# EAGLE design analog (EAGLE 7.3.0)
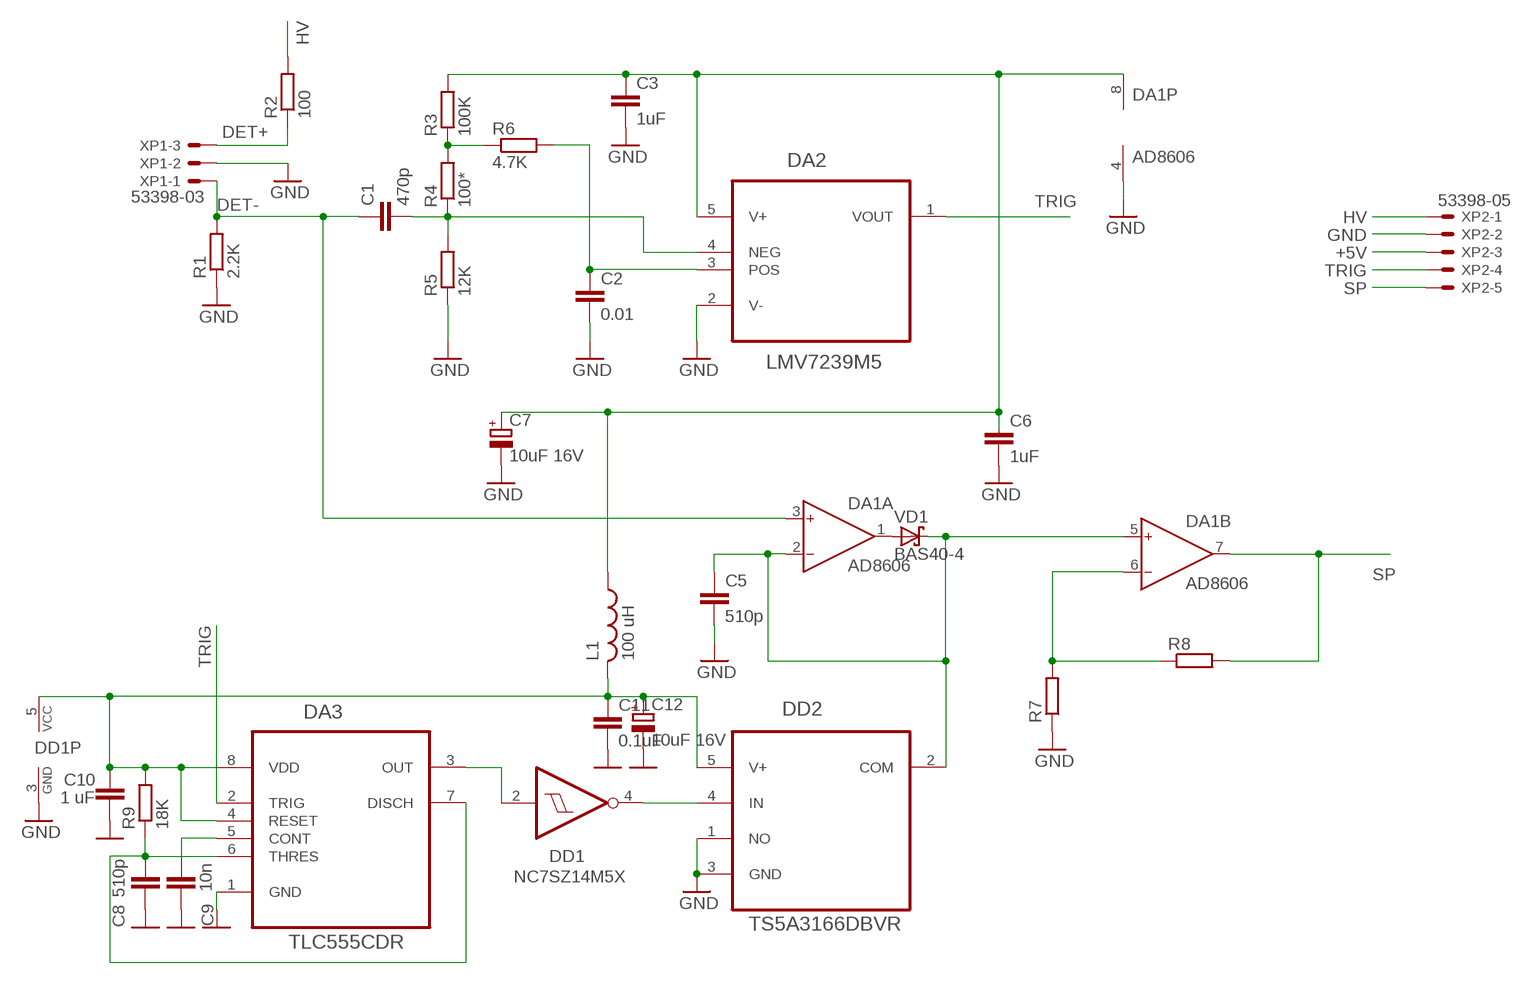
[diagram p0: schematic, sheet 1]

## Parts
C1  470p  C-EUC0603  [C0603]
C2  0.01  C-EUC0603  [C0603]
C3  1uF  C-EUC0805  [C0805]
C5  510p  C-EUC1206  [C1206]
C6  1uF  C-EUC0805  [C0805]
C7  10uF 16V  CPOL-EUSMCA  [SMC_A]
C8  510p  C-EUC0603K  [C0603K]
C9  10n  C-EUC0603K  [C0603K]
C10  1 uF  C-EUC0805  [C0805]
C11  0.1uF  C-EUC0805  [C0805]
C12  10uF 16V  CPOL-EUSMCA  [SMC_A]
DA1  AD8606  AD8607R  [SO8]
DA2  LMV7239M5  [SOT95P284X119-5N]
DA3  TLC555CDR  [SOIC127P600X175-8N]
DD1  NC7SZ14M5X  [SOT23-5]
DD2  TS5A3166DBVR  [SOT95P280X145-5N]
L1  100 uH  L-USL1812  [L1812]
R1  2.2K  R-EU_R0603  [R0603]
R2  100  R-EU_R0603  [R0603]
R3  100K  R-EU_R0603  [R0603]
R4  100*  R-EU_R0603  [R0603]
R5  12K  R-EU_R0603  [R0603]
R6  4.7K  R-EU_R0603  [R0603]
R7  R-EU_R0603  [R0603]
R8  R-EU_R0603  [R0603]
R9  18K  R-EU_R0603  [R0603]
VD1  BAS40-4  BAT54  [SOT23]
XP1  53398-03  [53398-03]
XP2  53398-05  [53398-05]

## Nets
+5V: C3.1 C6.1 C7.+ DA1.8(P:V+) DA2.5(V+) L1.1 R3.2 XP2.3
+5VD: C10.1 C11.1 C12.+ DA3.4(RESET) DA3.8(VDD) DD1.5(VCC) DD2.5(V+) L1.2 R9.2
DET+: R2.1 XP1.3
DET-: C1.1 DA1.3(A:IN+) R1.2 XP1.1
GND: C2.2 C3.2 C5.2 C6.2 C7.- C8.2 C9.2 C10.2 C11.2 C12.- DA1.4(P:V-) DA2.2(V-) DA3.1(GND) DD1.3(GND) DD2.1(NO) DD2.3(GND) R1.1 R5.1 R7.1 XP1.2 XP2.2
HV: R2.2 XP2.1
N$3: C1.2 DA2.4(NEG) R4.1 R5.2
N$4: R3.1 R4.2 R6.1
N$5: C2.1 DA2.3(POS) R6.2
N$7: DA1.1(A:OUT) VD1.1(A)
N$8: C5.1 DA1.2(A:IN-) DA1.5(B:IN+) DD2.2(COM) VD1.3(C)
N$9: DD1.4(O) DD2.4(IN)
N$10: DA3.3(OUT) DD1.2(I)
N$11: DA1.6(B:IN-) R7.2 R8.1
N$12: C9.1 DA3.5(CONT)
N$13: C8.1 DA3.6(THRES) DA3.7(DISCH) R9.1
SP: DA1.7(B:OUT) R8.2 XP2.5
TRIG: DA2.1(VOUT) DA3.2(TRIG) XP2.4

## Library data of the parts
C1-C3 C5 C6 C8-C11 = resistor:C-EU: CAPACITOR, European symbol
C7 C12 = resistor:CPOL-EU: POLARIZED CAPACITOR, European symbol
DA1 = analog-devices:AD8607: Precision Micropower, Low Noise CMOS, Rail-to-Rail Input/Output Operational Amplifiers Source: http://www.analog.com/static/imported-files/data_sheets/AD8603_8607_8609.pdf; MPN: AD8607ARMZ-R2; OC_FARNELL: 1651293; OC_NEWARK: 19M8927
DA2 = LMV7239M5:LMV7239M5: Comparator; AVAILABILITY: Good; DESCRIPTION: 75 nsec, Ultra Low Pwr, Low Voltage, Rail-to-Rail Input Comparator w/ Open-Drain/Push-Pull Output 5-SOT-23 -40 to 85; MF: Texas Instruments; MP: LMV7239M5; PACKAGE: SOT-23 Texas Instruments; PRICE: 1.72 USD
DA3 = Texas Instruments_By_element14_Batch_1:TLC555CDR: TIMER; MPN: TLC555CDR; OC_FARNELL: 8454426; OC_NEWARK: 35C2153; PACKAGE: SOIC-8; SUPPLIER: TI
DD1 = 74xx-little-us:NC7SZ14: TinyLogic(R) UHS Inverter with Schmitt Trigger Input Source: http://www.fairchildsemi.com/ds/NC/NC7SZ14.pdf
DD2 = Texas Instruments_By_element14_Batch_1:TS5A3166DBVR: .9- OHM SPST ANALOG SWITCH; MPN: TS5A3166DBVR; OC_FARNELL: 1755409; OC_NEWARK: 08K5004; PACKAGE: SOT-23-5; SUPPLIER: Texas Instruments
L1 = resistor:L-US: INDUCTOR, American symbol
R1-R9 = resistor:R-EU_: RESISTOR, European symbol
VD1 = diode:BAT54: Schottky Diodes
XP1 = con-molex:53?-03: CONNECTOR wire to board 1.25 mm (.049 inch) pitch header; OC_FARNELL: unknown; OC_NEWARK: unknown
XP2 = con-molex:53?-05: CONNECTOR wire to board 1.25 mm (.049 inch) pitch header; OC_FARNELL: 1125354; OC_NEWARK: unknown

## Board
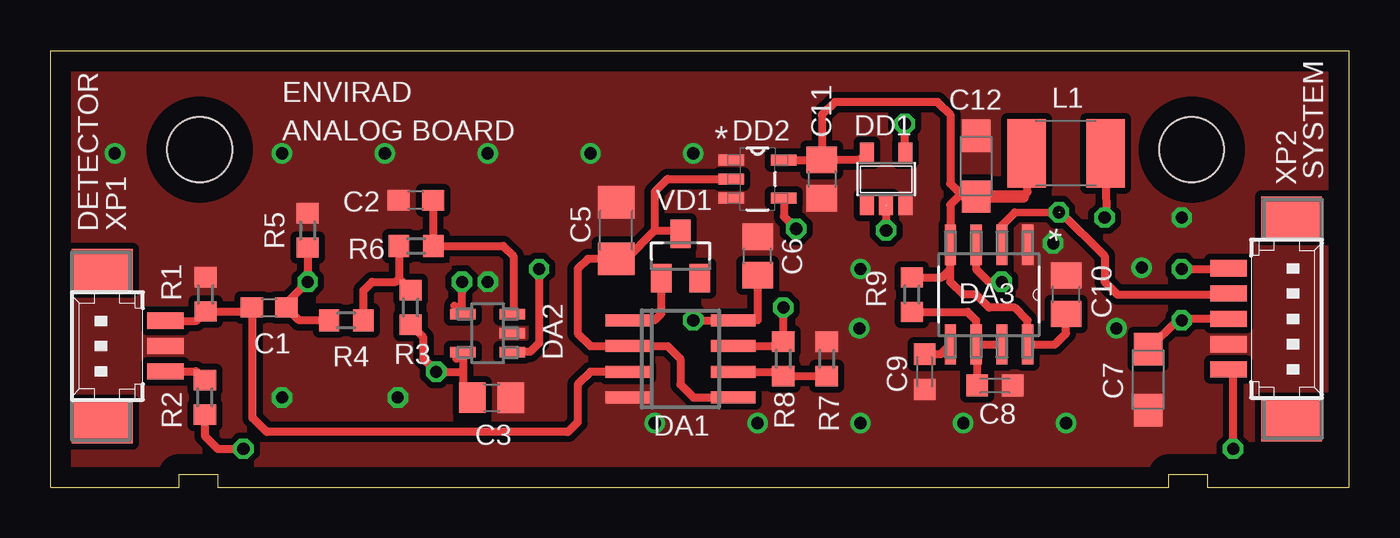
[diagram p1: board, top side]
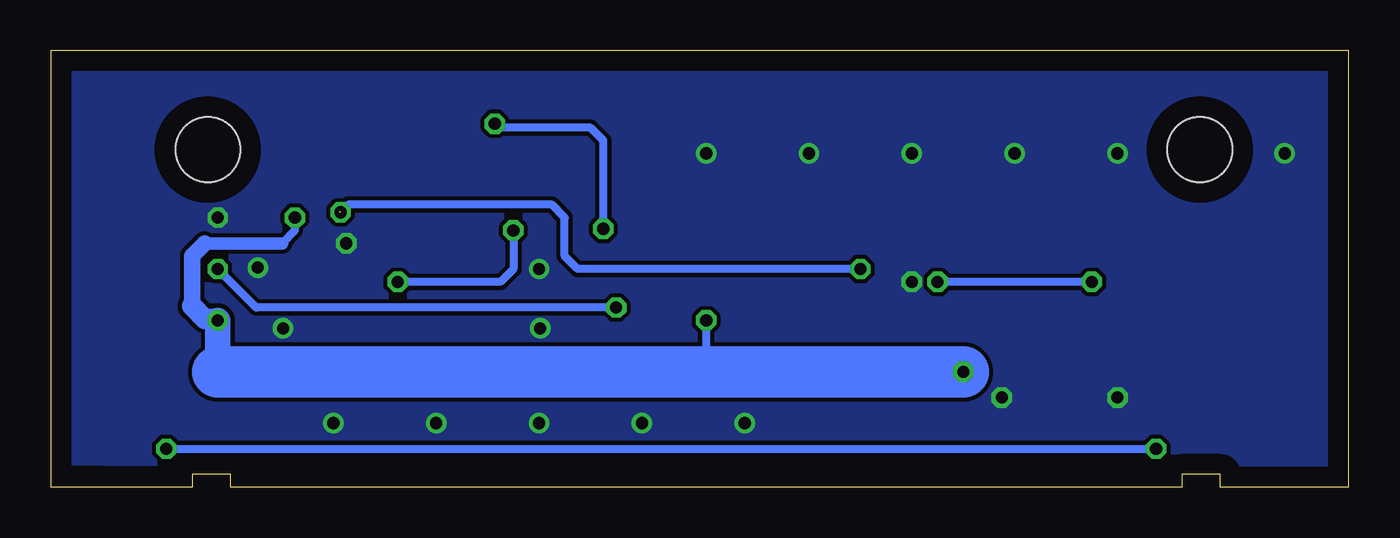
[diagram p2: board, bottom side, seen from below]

Size 64.13 x 21.59 mm. Coordinates in mm from the lower left corner, seen from the top.
Outline: 0,21.59 64.13,21.59 64.13,0 57.15,0 57.15,0.63 55.25,0.63 55.25,0 8.26,0 8.26,0.63 6.35,0.63 6.35,0 0,0 0,21.59
Copper layers (1*16): Top 0.035mm / dielectric 1.5mm / Bottom 0.035mm
Design rules "default *": minimum track width 8mil, minimum drill 12mil, track to track 8mil, track to pad 8mil, pad to pad 8mil, via to via 8mil, smd to smd 8mil, copper to edge 40mil, drill to drill 8mil, minimum pad ring 10mil, minimum via ring 8mil, stop-mask expansion 4mil, vias tented up to drill 32mil, thermal gap 10mil
Holes 3.2 mm at 7.37,16.7 56.37,16.7

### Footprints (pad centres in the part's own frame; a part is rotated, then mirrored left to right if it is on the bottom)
C0603 = smd 1.1 x 1: 1 -0.85,0; 2 0.85,0
C0805 = smd 1.3 x 1.5: 1 -0.95,0; 2 0.95,0
C1206 = smd 1.6 x 1.8: 1 -1.4,0; 2 1.4,0
SMC_A = smd 1.6 x 1.4: + -1.5,0; - 1.5,0
C0603K = smd 1.05 x 1.08: 1 -0.875,0; 2 0.875,0
SO8 = smd 0.6 x 2.2: 1 -1.905,-2.6; 2 -0.635,-2.6; 3 0.635,-2.6; 4 1.905,-2.6; 5 1.905,2.6; 6 0.635,2.6; 7 -0.635,2.6; 8 -1.905,2.6
SOT95P284X119-5N = smd 1.27 x 0.533: 1 -1.219,0.94; 2 -1.219,0; 3 -1.219,-0.94; 4 1.219,-0.94; 5 1.219,0.94
SOIC127P600X175-8N = smd 1.981 x 0.559: 1 -2.464,1.905; 2 -2.464,0.635; 3 -2.464,-0.635; 4 -2.464,-1.905; 5 2.464,-1.905; 6 2.464,-0.635; 7 2.464,0.635; 8 2.464,1.905
SOT23-5 = smd 0.69 x 0.99: 1 -0.95,-1.29; 2 0,-1.29; 3 0.95,-1.29; 4 0.95,1.3; 5 -0.95,1.3
SOT95P280X145-5N = smd 1.27 x 0.559: 1 -1.295,0.94; 2 -1.295,0; 3 -1.295,-0.94; 4 1.295,-0.94; 5 1.295,0.94
L1812 = smd 1.9 x 3.4: 1 -1.95,0; 2 1.95,0
R0603 = smd 1 x 1.1: 1 -0.85,0; 2 0.85,0
SOT23 = smd 1 x 1.4: 1 -0.95,-1.1; 2 0.95,-1.1; 3 0,1.1
53398-03 = smd 0.8 x 1.8: 1 1.25,-2.5; 2 0,-2.5; 3 -1.25,-2.5 | smd 2.1 x 3: S1 3.75,0.625; S2 -3.75,0.625
53398-05 = smd 0.8 x 1.8: 1 2.5,-2.5; 2 1.25,-2.5; 3 0,-2.5; 4 -1.25,-2.5; 5 -2.5,-2.5 | smd 2.1 x 3: S1 5,0.625; S2 -5,0.625

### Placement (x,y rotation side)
C1  10.79,8.89 0 top
C2  18.04,14.19 180 top
C3  21.79,4.44 0 top
C5  27.94,12.7 90 top
C6  34.93,11.43 90 top
C7  54.21,5.33 270 top
C8  46.65,5.03 0 top
C9  43.18,5.71 270 top
C10  50.16,9.52 90 top
C11  38.1,15.24 270 top
C12  45.72,15.88 90 top
DA1  31.11,6.35 270 top
DA2  21.59,7.62 180 top
DA3  46.36,9.52 270 top
DD1  41.27,15.24 0 top
DD2  34.93,15.24 0 top
L1  50.16,16.51 180 top
R1  7.65,9.54 270 top
R2  7.62,4.45 270 top
R3  17.78,8.89 270 top
R4  14.61,8.25 0 top
R5  12.7,12.7 270 top
R6  18.06,11.93 0 top
R7  38.34,6.35 270 top
R8  36.2,6.35 90 top
R9  42.55,9.52 90 top
VD1  31.11,11.43 0 top
XP1  3.17,6.98 90 top
XP2  60.68,8.33 270 top

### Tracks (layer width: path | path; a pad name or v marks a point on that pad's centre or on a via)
+5V  (via drill 0.6)
  Top 0.406: 20.04,6.35 DA2.5 20.37,5.71 | 20.37,5.71 20.37,4.91 C3.1 | C6.1 34.93,8.25 DA1.8 v31.75,8.25 | XP2.3 55.81,8.33 | C7.+ 55.72,8.33 55.81,8.33 | L1.1 52.16,13.43 v52.07,13.34 | 20.37,5.71 v19.05,5.71 18.41,6.35 18.41,7.41 R3.2 | 55.81,8.33 v55.88,8.25
  Bottom 0.406: v52.07,13.34 52.07,12.7 52.71,12.06 | 55.95,8.33 v55.88,8.25 | v31.75,8.25 31.75,5.71
  Bottom 0.61: 52.71,12.06 56.52,12.06
  Bottom 0.813: 56.52,12.06 57.15,11.43 57.15,8.96
  Bottom 1.016: 57.15,8.96 56.52,8.33 55.95,8.33
  Bottom 1.27: v55.88,8.25 55.88,5.71
  Bottom 2.54: 55.88,5.71 31.75,5.71 v19.05,5.71
+5VD
  Top 0.406: C12.+ 45.09,14.38 | 45.09,14.38 44.86,14.38 44.45,13.97 DA3.4 44.45,10.79 | R9.2 44.03,10.38 44.45,10.79 | C10.1 50.16,7.62 49.61,7.06 DA3.8 48.26,8.25 47.62,8.89 46.36,8.89 45.72,9.52 45.09,9.52 44.45,10.16 44.45,10.79 | 45.09,14.38 44.45,15.01 44.45,18.41 43.82,19.05 38.73,19.05 38.1,18.41 C11.1 | DD2.5 C11.1 | C11.1 39.98,16.19 DD1.5 | 48.03,14.38 48.26,14.6 48.26,15.78 L1.2
  Top 0.61: C12.+ 48.03,14.38
DET+
  Top 0.406: XP1.3 7.18,5.73 R2.1
DET-
  Top 0.406: XP1.1 7.2,8.23 R1.2 9.75,8.69 C1.1 9.98,8.86 9.98,3.43 10.68,2.73 25.55,2.73 26.04,3.22 26.04,5.08 26.67,5.71 DA1.3
GND  (via drill 0.6)
  other vias: 3.17,16.51 11.43,4.45 49.53,12.06 21.59,10.16 11.43,16.51 16.51,16.51 21.59,16.51 26.67,16.51 31.75,16.51 29.84,3.17 34.93,3.17 40.01,3.17 45.09,3.17 50.16,3.17 40.01,10.79 39.95,7.86 52.65,7.86 53.9,10.86 55.88,13.34 17.14,4.45
  pour Bottom: 0,20.95 0,0.63 64.13,1.27 64.13,20.95
  pour Top (isolate 0.305, no thermals): 0,20.95 64.13,20.95 64.13,1.27 0,0.63
HV  (via drill 0.6)
  Top 0.406: v58.42,1.91 58.42,5.59 XP2.1 | R2.2 7.62,2.54 8.26,1.91 v9.53,1.91
  Bottom 0.406: v58.42,1.91 v9.53,1.91
N$3  (via drill 0.6)
  Top 0.406: 19.95,8.98 20.18,8.75 | 20.18,8.75 DA2.4 | v20.32,10.16 20.32,8.89 20.18,8.75 | R5.2 v12.7,10.16 11.43,8.89 C1.2 12.28,8.25 R4.1
  Bottom 0.406: v12.7,10.16 v20.32,10.16
N$4
  Top 0.406: R6.1 17.21,10.31 | 17.21,10.31 R3.1 | R4.2 15.46,9.74 15.88,10.16 17.05,10.16 17.21,10.31
N$5
  Top 0.406: C2.1 18.89,11.95 R6.2 22.36,11.93 22.86,11.43 22.86,8.61 DA2.3
N$7
  Top 0.406: VD1.1 30.16,8.57 29.84,8.25 DA1.1
N$8
  Top 0.406: DA1.5 31.75,4.45 31.11,5.08 31.11,6.35 30.48,6.98 DA1.2 26.67,6.98 26.04,7.62 26.04,10.79 26.54,11.3 C5.1 28.44,11.3 29.84,12.7 | 29.84,12.7 30.94,12.7 VD1.3 | 29.84,12.7 29.84,14.6 30.48,15.24 DD2.2
N$9  (via drill 0.6)
  Top 0.406: v42.19,17.97 42.19,16.57 DD1.4 | DD2.4 36.22,13.39 v36.83,12.78
  Bottom 0.406: v36.83,12.78 36.83,17.15 37.47,17.78 42,17.78 v42.19,17.97
N$10  (via drill 0.6)
  Top 0.406: DA3.3 45.72,10.79 46.36,10.16 v46.99,10.16 | DD1.2 v41.27,12.7
  Bottom 0.406: v41.27,12.7 41.27,10.79 41.91,10.16 v46.99,10.16
N$11
  Top 0.406: DA1.6 35.98,5.71 R8.1 R7.2
N$12
  Top 0.406: C9.1 43.98,6.59 DA3.5
N$13
  Top 0.406: DA3.6 DA3.7 | C8.1 45.77,7.01 DA3.6 | R9.1 45.3,8.67 45.72,8.25 DA3.6
SP  (via drill 0.6)
  Top 0.406: DA1.7 35.98,6.98 R8.2 v36.2,8.89 | v55.88,10.79 58.15,10.79 XP2.5
  Bottom 0.406: v36.2,8.89 53.98,8.89 v55.88,10.79
TRIG  (via drill 0.6)  (1 unrouted)
  Top 0.406: XP2.4 58.13,9.52 52.71,9.52 52.07,10.16 52.07,11.43 49.88,13.6 47.62,13.59 46.99,12.95 DA3.2 | v24.13,10.79 24.13,7.14 23.69,6.7 22.83,6.7 DA2.1
  Bottom 0.406: v24.13,10.79 38.1,10.79 38.73,11.43 38.73,13.34 39.37,13.97 49.44,13.97 v49.81,13.6

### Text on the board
tNames: ENVIRAD | ANALOG BOARD | DD2 | SYSTEM | DETECTOR | C1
